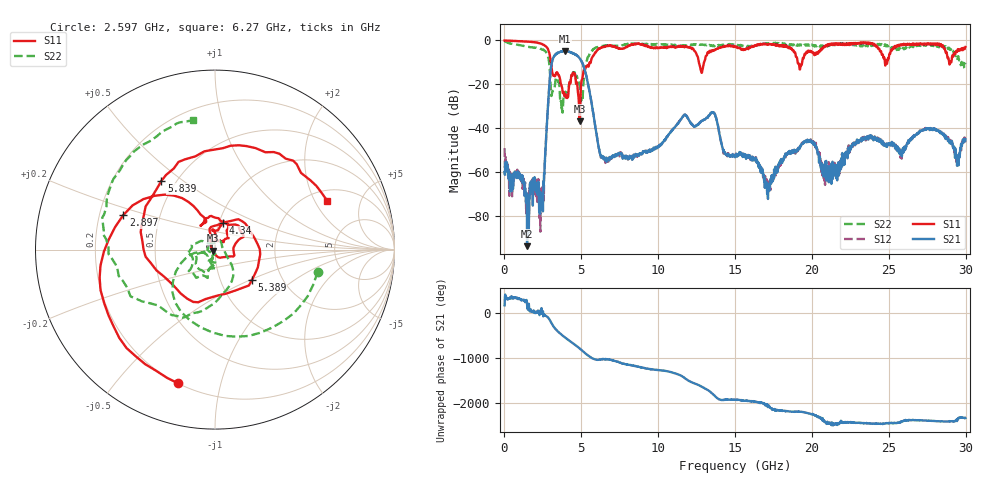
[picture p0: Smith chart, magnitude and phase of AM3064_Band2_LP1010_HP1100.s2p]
# Hz S DB R 50.0
!freq dBS11 angS11 dBS21 angS21 dBS12 angS12 dBS22 angS22
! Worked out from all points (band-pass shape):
!   1600 points, 10 MHz to 29.98 GHz, reference 50 ohm
!   highest |S21| = -4.86 dB at 3.927 GHz (marker M1); lowest = -93.5 dB at 1.472 GHz (marker M2)
!   |S21| within 3 dB of the highest: 3.181 GHz to 4.863 GHz (1.682 GHz wide, 41.8 % of centre)
!   lowest |S11| = -36.8 dB at 4.883 GHz (marker M3), VSWR 1.03, Z = 48.7 - j0.66 ohm
!   |S11| at or under -10 dB: 3.021 GHz to 5.61 GHz (2.589 GHz wide, 60 % of centre); 12.64 GHz to 12.98 GHz (337 MHz wide, 2.63 % of centre); 19.07 GHz to 19.36 GHz (290.7 MHz wide, 1.51 % of centre)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
!   |S22| runs from -32.8 to -0.3 dB; largest |S21 - S12| = 0.014
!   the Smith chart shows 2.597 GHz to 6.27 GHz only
!   S11 on the Smith chart (normalised r, x): 2.597 GHz: 0.20, -0.74; 2.897 GHz: 0.30, +0.17; 4.34 GHz: 1.04, +0.31; 5.389 GHz: 1.41, -0.51; 5.839 GHz: 0.42, +0.42; 6.27 GHz: 2.49, +2.54
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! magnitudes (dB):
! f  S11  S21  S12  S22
! 10 MHz  0.0  -59.8  -49.0  -0.3
! 1.472 GHz  -0.6  -93.5  -70.4  -2.9
! 2.409 GHz  -1.6  -72.3  -74.5  -4.0
! 2.597 GHz  -2.2  -60.6  -58.9  -4.7
! 2.897 GHz  -5.3  -22.7  -22.7  -9.5
! 3.196 GHz  -15.9  -7.7  -7.6  -22.9
! 3.927 GHz  -25.2  -4.9  -4.8  -25.3
! 4.34 GHz  -16.3  -5.7  -5.5  -16.1
! 4.883 GHz  -36.8  -8.0  -8.1  -20.3
! 5.015 GHz  -18.4  -9.6  -9.5  -26.0
! 5.389 GHz  -11.5  -18.3  -18.1  -8.4
! 5.839 GHz  -6.3  -36.0  -35.8  -3.8
! 6.27 GHz  -3.3  -52.2  -53.3  -2.7
! 10 GHz  -3.4  -48.2  -48.1  -1.9
! 12.81 GHz  -14.6  -36.7  -36.7  -2.0
! 13.54 GHz  -4.9  -32.7  -32.5  -2.6
! 15 GHz  -2.7  -53.2  -51.8  -1.8
! 17.09 GHz  -1.7  -69.7  -65.9  -1.5
! 19.99 GHz  -5.1  -46.4  -46.1  -1.9
! 20.82 GHz  -2.9  -56.2  -63.9  -2.3
! 25 GHz  -8.0  -46.9  -46.9  -2.3
! 29.98 GHz  -3.0  -44.9  -46.4  -10.1
